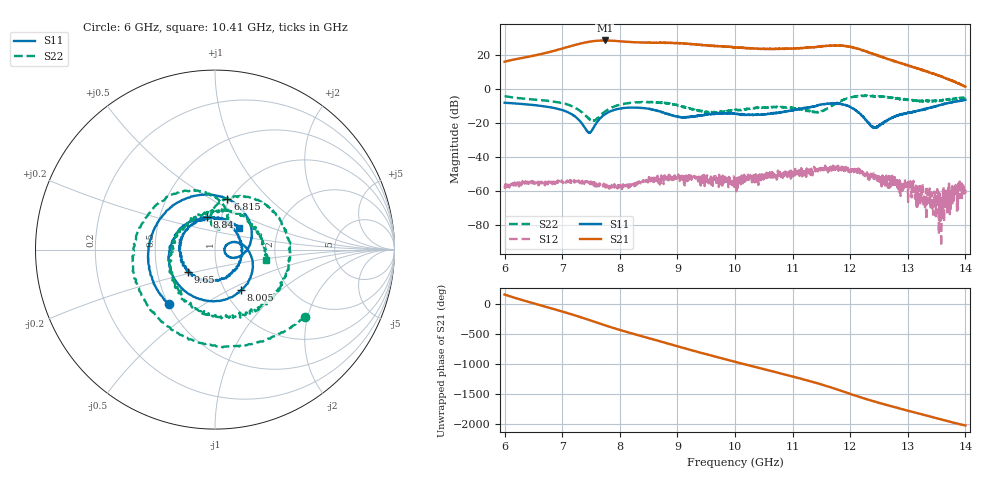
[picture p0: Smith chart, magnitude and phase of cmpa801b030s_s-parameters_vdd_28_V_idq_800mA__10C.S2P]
!Keysight Technologies,E5071C,MY46110325,B.14.03
!Date: Fri Aug 07 13:44:56 2020
!Data & Calibration Information:
!Freq	S11:SOLT2(ON)	S21:SOLT2(ON)	S12:SOLT2(ON)	S22:SOLT2(ON)
!PortZ  Port1:50+j0  Port2:50+j0
!Above PortZ is port z conversion or system Z0 setting when saving the data.
!When reading, reference impedance value at option line is always used.
# Hz S dB R 50
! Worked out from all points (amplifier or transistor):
!   1601 points, 6 GHz to 14 GHz, reference 50 ohm
!   highest |S21| = 28.7 dB at 7.74 GHz (marker M1)
!   |S21| within 3 dB of that: 7.182 GHz to 9.53 GHz (2.348 GHz wide, 28.1 % of centre)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
!   unconditionally stable (mu >= 1): start of sweep to end of sweep
!   at 7.33 GHz: K = 11.38, MAG = 27.2 dB, |S12| = -54.5 dB
!   at 10 GHz: K = 12.27, MAG = 25.0 dB, |S12| = -53.2 dB
!   at 14 GHz: K = 190.55, MAG = 4.6 dB, |S12| = -59.2 dB
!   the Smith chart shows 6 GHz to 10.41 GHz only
!   S11 on the Smith chart (normalised r, x): 6 GHz: 0.50, -0.36; 6.815 GHz: 0.97, +0.60; 8.005 GHz: 1.19, -0.58; 8.84 GHz: 0.85, +0.33; 9.65 GHz: 0.72, -0.19; 10.41 GHz: 1.26, +0.32
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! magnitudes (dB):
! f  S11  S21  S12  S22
! 6 GHz  -8.0  16.2  -56.6  -4.0
! 6.815 GHz  -10.7  22.2  -54.6  -7.1
! 7.335 GHz  -19.9  27.0  -55.2  -13.4
! 7.48 GHz  -25.6  28.0  -55.4  -17.8
! 7.74 GHz  -14.8  28.7  -56.5  -13.2
! 8.005 GHz  -11.4  28.1  -56.7  -9.1
! 8.67 GHz  -12.9  27.3  -52.4  -7.8
! 8.84 GHz  -14.4  27.4  -52.4  -8.4
! 9.65 GHz  -14.1  25.3  -51.4  -13.6
! 10 GHz  -14.4  24.6  -53.2  -12.2
! 10.41 GHz  -14.9  23.8  -52.4  -10.7
! 11.34 GHz  -10.4  24.6  -47.1  -13.2
! 11.94 GHz  -9.6  25.2  -46.5  -5.5
! 12.41 GHz  -22.6  20.7  -50.7  -4.1
! 12.67 GHz  -17.8  17.7  -52.2  -4.7
! 13.06 GHz  -13.8  13.2  -60.7  -6.5
! 13.15 GHz  -12.8  12.3  -60.7  -6.8
! 13.22 GHz  -12.4  11.5  -60.9  -6.8
! 13.3 GHz  -11.6  10.7  -69.4  -6.9
! 13.56 GHz  -9.3  7.7  -77.5  -6.7
! 13.8 GHz  -7.4  4.6  -65.7  -5.7
! 14 GHz  -6.2  1.6  -59.2  -4.6
